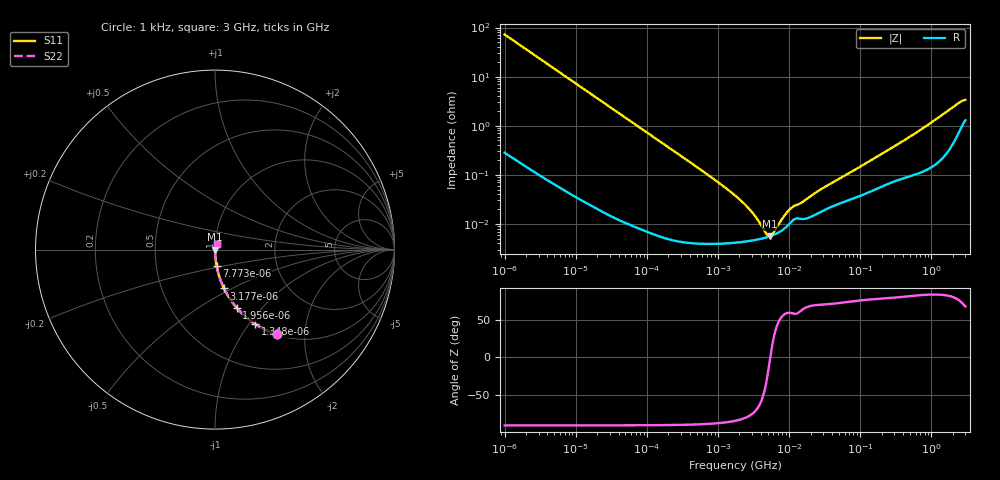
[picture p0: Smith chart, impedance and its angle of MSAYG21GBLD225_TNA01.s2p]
! MSAYG21GBLD225_TNA01  S-PARAMETER MODEL  ( Standard Model )
! Model Generated by TAIYO YUDEN Corporation (http://www.ty-top.com)
! Version 1.0
! TAIYO YUDEN Control No. 220601
! Copyright(c) 2012 TAIYO YUDEN CO.,LTD. All Rights Reserved.
! Product Description (link to TY-COMPAS)
! https://ds.yuden.co.jp/TYCOMPAS/or/detail?pn=MSAYG21GBLD225KTNA01&u=M
! Products Name : Multilayer Ceramic Capacitors
! Characteristics :
!  Capacitance : 2.2 [uF] , Rated Voltage : 35 [V] , TCC : X5R
!  Case Size : 2.0 x 1.25 / 0.079 x 0.049 [mm/inch] , Thickness : 1.25 / 0.049 [mm/inch]
!  (Conditions: Temperature = 25 [degC] , DC Bias Voltage = 0 [V])
! External Node Assignments :
!  1  o---| |---o  2
! GND o---------o GND
! Frequency Range : 1kHz  -  3GHz  [ 401 STEP ]
# MHZ S RI R 50
! Freq[MHz].  S11 Real  S11 Imag  S21 Real  S21 Imag  S12 Real  S12 Imag  S22 Real  S22 Imag
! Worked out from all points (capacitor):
!   401 points, 1 kHz to 3 GHz, reference 50 ohm
!   read as one part in series: C = 2.2 uF near 1.077 kHz
!   lowest |Z| = 5.6 mohm at 5.301 MHz (marker M1)
!   series resonance near 5.429 MHz, so ESL is about 390 pH
!   S11 on the Smith chart (normalised r, x): 1 kHz: 1.01, -1.44; 1.348 kHz: 1.00, -1.07; 1.956 kHz: 1.00, -0.74; 3.177 kHz: 1.00, -0.46; 7.773 kHz: 1.00, -0.19; 3 GHz: 1.03, +0.06
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0.001  0.3429 -0.4728  0.6571 0.4728  0.6571 0.4728  0.3429 -0.4728
0.001348  0.224 -0.4149  0.776 0.4149  0.776 0.4149  0.224 -0.4149
0.001956  0.1211 -0.3242  0.8789 0.3242  0.8789 0.3242  0.1211 -0.3242
0.003177  0.0502 -0.2162  0.9498 0.2162  0.9498 0.2162  0.0502 -0.2162
0.007773  0.00906 -0.0924  0.9909 0.0924  0.9909 0.0924  0.00906 -0.0924
0.01216  0.00385 -0.0595  0.9961 0.0595  0.9961 0.0595  0.00385 -0.0595
0.147855  8.04e-05 -0.00495  0.9999 0.00495  0.9999 0.00495  8.04e-05 -0.00495
0.762639  4e-05 -0.000941  1 0.000941  1 0.000941  4e-05 -0.000941
1.732051  4.15e-05 -0.000378  1 0.000378  1 0.000378  4.15e-05 -0.000378
2.610246  4.44e-05 -0.000213  1 0.000213  1 0.000213  4.44e-05 -0.000213
3.93371  4.93e-05 -8.71e-05  1 8.71e-05  1 8.71e-05  4.93e-05 -8.71e-05
4.238263  5.06e-05 -6.64e-05  0.9999 6.64e-05  0.9999 6.64e-05  5.06e-05 -6.64e-05
5.30084  5.56e-05 -6.3e-06  0.9999 6.3e-06  0.9999 6.3e-06  5.56e-05 -6.3e-06
6.629817  6.35e-05 5.31e-05  0.9999 -5.31e-05  0.9999 -5.31e-05  6.35e-05 5.31e-05
7.143107  6.72e-05 7.32e-05  0.9999 -7.32e-05  0.9999 -7.32e-05  6.72e-05 7.32e-05
10.76485  0.000111 0.000182  0.9999 -0.000182  0.9999 -0.000182  0.000111 0.000182
15.05716  0.000126 0.000242  0.9999 -0.000242  0.9999 -0.000242  0.000126 0.000242
21.06097  0.000143 0.000362  0.9999 -0.000362  0.9999 -0.000362  0.000143 0.000362
256.0921  0.00068 0.00324  0.9993 -0.00324  0.9993 -0.00324  0.00068 0.00324
727.4359  0.0012 0.00844  0.9988 -0.00844  0.9988 -0.00844  0.0012 0.00844
2398.636  0.00771 0.0275  0.9923 -0.0275  0.9923 -0.0275  0.00771 0.0275
3000  0.0137 0.03  0.9863 -0.03  0.9863 -0.03  0.0137 0.03
